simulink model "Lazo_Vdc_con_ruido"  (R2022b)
settings: Solver=ode4  StartTime=0.0  StopTime=0.2  FixedStep=1e-6  RelTol=1e-3
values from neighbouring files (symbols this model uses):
  C_DC = 6.8e-3    (= 0.0068)    [PI_Lazo_V_DC.m]    (also in LQR_Sin_Integral.m; LQR_Con_Integral.m; Modal_Integral.m; Sistema_no_lineal_Modal.m)
  Delta_I_DC_2 = -2*I_DC0_2    (= 12)    [PI_Lazo_V_DC.m]
  i_d0_1 = 14.14213562    [PI_Lazo_V_DC.m]    (also in Sistema_no_lineal_Modal.m = ((3000*2)/(3*v_d_1))*1.06522; Sistema_no_lineal_LQR.m = ((3000*2)/(3*v_d_1))*1.06522; Sistema_control_no_lineal_LQR.m = ((3000*2)/(3*v_d_1))*1.06522; Sistema_control_no_lineal_Modal.m = ((3000*2)/(3*v_d_1))*1.06522)
  I_DC0_2 = -6    [PI_Lazo_V_DC.m]
  Ki_DC = q_12/q_22    [PI_Lazo_V_DC.m]    (also in Sistema_control_no_lineal_LQR.m; Sistema_control_no_lineal_Modal.m)
  Kp_DC = q_11/q_21    [PI_Lazo_V_DC.m]    (also in Sistema_control_no_lineal_LQR.m; Sistema_control_no_lineal_Modal.m)
  lim_i_d_1_lower = -75.07117    [PI_Lazo_V_DC.m]    (also in Sistema_control_no_lineal_LQR.m; Sistema_control_no_lineal_Modal.m)
  lim_i_d_1_upper = 75.07117    [PI_Lazo_V_DC.m]    (also in Sistema_control_no_lineal_LQR.m; Sistema_control_no_lineal_Modal.m)
  v_d_1 = 100*sqrt(2)    [PI_Lazo_V_DC.m]    (also in LQR_Sin_Integral.m; LQR_Con_Integral.m; Modal_Integral.m; Sistema_no_lineal_Modal.m)
  V_DC0 = 500    [PI_Lazo_V_DC.m]    (also in LQR_Sin_Integral.m; LQR_Con_Integral.m; Modal_Integral.m; Sistema_no_lineal_Modal.m)
  V_R_V = D_R_V^2    (= 0.0009)    [PI_Lazo_V_DC.m]    (also in Sistema_no_lineal_Modal.m = 4e-06; Sistema_no_lineal_LQR.m = 4e-06; Sistema_control_no_lineal_LQR.m; Sistema_control_no_lineal_Modal.m)
undefined symbols (not defined in the file or in its folder): V_v_d_1, V_V_DC

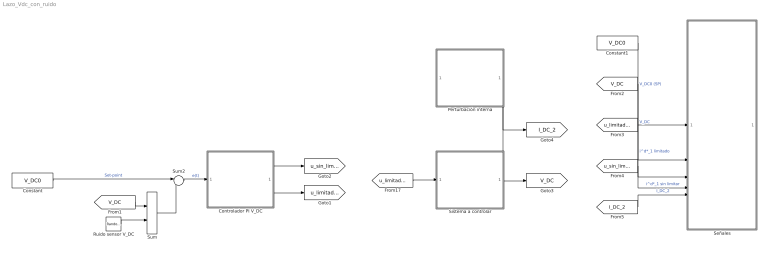
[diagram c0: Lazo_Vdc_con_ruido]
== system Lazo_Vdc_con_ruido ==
  Constant : Constant  Value=V_DC0
  Constant1 : Constant  Value=V_DC0
  Controlador PI V_DC : Subsystem
  Perturbación interna : Subsystem
  Ruido sensor V_DC : RandomNumber  Variance=V_R_V  SampleTime=0.001
  Señales : Subsystem
  Sistema a controlar : Subsystem
  Sum : Sum
  Sum2 : Sum  Inputs=|+-
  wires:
  Constant/1 -> Sum2/1  "Set-point"
  Sum2/1 -> Controlador PI V_DC/1(e(t))  "e(t)"
  Controlador PI V_DC/2(i^d*_1 limitado) -> [u_limitado_1]
  Perturbación interna/1(I_DC_2) -> [I_DC_2], Sistema a controlar/2(I_DC_2)
  Controlador PI V_DC/1(i^d*_1 sin limitar) -> [u_sin_limitar_1]
  [u_limitado_1] -> Sistema a controlar/1(i^d*_1 limitado)
  Sistema a controlar/1(V_DC) -> [V_DC]
  Constant1/1 -> Señales/1(V_DC0 (SP))  "V_DC0 (SP)"
  [V_DC] -> Señales/2(V_DC1)  "V_DC"
  [u_limitado_1] -> Señales/3(i^d*_1 limitado)  "i^d*_1 limitado"
  [u_sin_limitar_1] -> Señales/4(i^d*_1 sin limitar)  "i^d*_1 sin limitar"
  [I_DC_2] -> Señales/5(I_DC_2)  "I_DC_2"
  [V_DC] -> Sum/1
  Ruido sensor V_DC/1 -> Sum/2
  Sum/1 -> Sum2/2

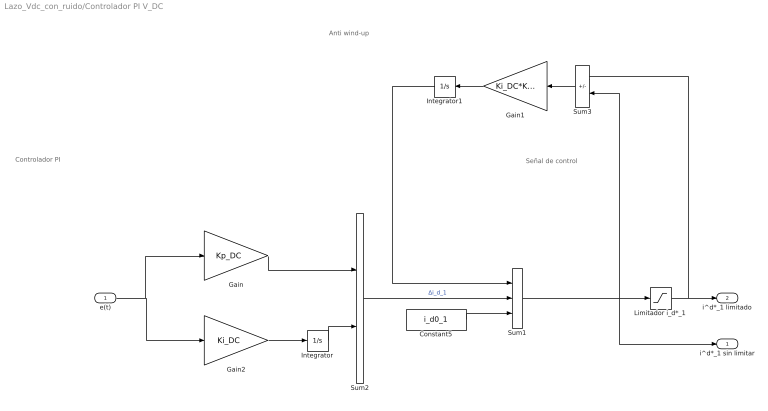
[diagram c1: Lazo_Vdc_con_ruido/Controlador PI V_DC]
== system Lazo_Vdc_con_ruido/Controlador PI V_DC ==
  note: Señal de control
  note: Controlador PI
  note: Anti wind-up
  e(t) : Inport
  Constant5 : Constant  Value=i_d0_1
  Gain : Gain  Gain=Kp_DC
  Gain1 : Gain  Gain=Ki_DC*Ki_DC
  Gain2 : Gain  Gain=Ki_DC
  Integrator : Integrator
  Integrator1 : Integrator
  Limitador i_d*_1 : Saturate  UpperLimit=lim_i_d_1_upper  LowerLimit=lim_i_d_1_lower
  Sum1 : Sum  Inputs=+++
  Sum2 : Sum
  Sum3 : Sum  Inputs=+-
  i^d*_1 sin limitar : Outport
  i^d*_1 limitado : Outport  Port=2
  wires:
  Limitador i_d*_1/1 -> Sum3/1, i^d*_1 limitado/1
  Constant5/1 -> Sum1/3
  Sum1/1 -> i^d*_1 sin limitar/1, Sum3/2, Limitador i_d*_1/1
  Sum2/1 -> Sum1/2  "Δi_d_1"
  Gain2/1 -> Integrator/1
  Integrator/1 -> Sum2/2
  Gain/1 -> Sum2/1
  e(t)/1 -> Gain/1, Gain2/1
  Sum3/1 -> Gain1/1
  Gain1/1 -> Integrator1/1
  Integrator1/1 -> Sum1/1

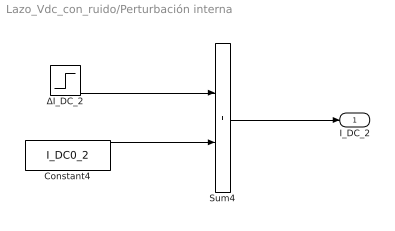
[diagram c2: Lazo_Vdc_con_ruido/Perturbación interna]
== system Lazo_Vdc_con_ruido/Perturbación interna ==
  Constant4 : Constant  Value=I_DC0_2
  Sum4 : Sum
  ΔI_DC_2 : Step  Time=0.05  After=Delta_I_DC_2  SampleTime=0
  I_DC_2 : Outport
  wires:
  ΔI_DC_2/1 -> Sum4/1
  Sum4/1 -> I_DC_2/1
  Constant4/1 -> Sum4/2

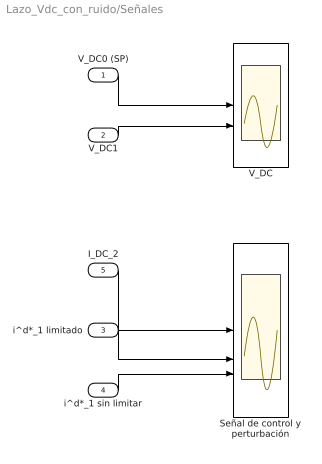
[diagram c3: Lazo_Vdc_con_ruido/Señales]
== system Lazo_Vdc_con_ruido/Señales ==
  V_DC0 (SP) : Inport
  V_DC1 : Inport  Port=2
  i^d*_1 limitado : Inport  Port=3
  i^d*_1 sin limitar : Inport  Port=4
  I_DC_2 : Inport  Port=5
  Señal de control y perturbación : Scope  NumInputPorts=3
  V_DC : Scope  NumInputPorts=2
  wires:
  I_DC_2/1 -> Señal de control y perturbación/1
  V_DC0 (SP)/1 -> V_DC/1
  i^d*_1 sin limitar/1 -> Señal de control y perturbación/3
  i^d*_1 limitado/1 -> Señal de control y perturbación/2
  V_DC1/1 -> V_DC/2

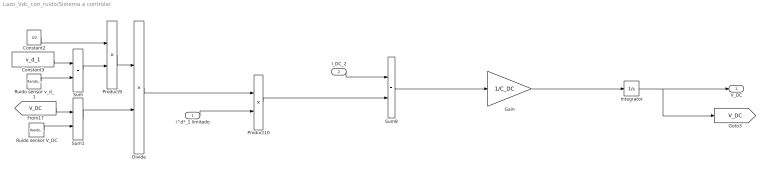
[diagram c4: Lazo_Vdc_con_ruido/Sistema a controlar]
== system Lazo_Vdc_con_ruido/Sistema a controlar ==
  i^d*_1 limitado : Inport
  I_DC_2 : Inport  Port=2
  Constant2 : Constant  Value=3/2
  Constant3 : Constant  Value=v_d_1
  Divide : Product  Inputs=*/
  Gain : Gain  Gain=1/C_DC
  Integrator : Integrator  InitialCondition=V_DC0
  Product10 : Product
  Product9 : Product
  Ruido sensor V_DC : RandomNumber  Commented=on  Variance=V_V_DC  SampleTime=0.001
  Ruido sensor v_d_1 : RandomNumber  Commented=on  Variance=V_v_d_1  SampleTime=0.001
  Sum : Sum
  Sum1 : Sum
  Sum8 : Sum
  V_DC : Outport
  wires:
  Gain/1 -> Integrator/1
  Divide/1 -> Product10/1
  I_DC_2/1 -> Sum8/1
  i^d*_1 limitado/1 -> Product10/2
  Sum8/1 -> Gain/1
  Integrator/1 -> [V_DC], V_DC/1
  Product10/1 -> Sum8/2
  [V_DC] -> Sum1/1
  Constant3/1 -> Sum/1
  Product9/1 -> Divide/1
  Constant2/1 -> Product9/1
  Sum/1 -> Product9/2
  Ruido sensor v_d_1/1 -> Sum/2
  Ruido sensor V_DC/1 -> Sum1/2
  Sum1/1 -> Divide/2
